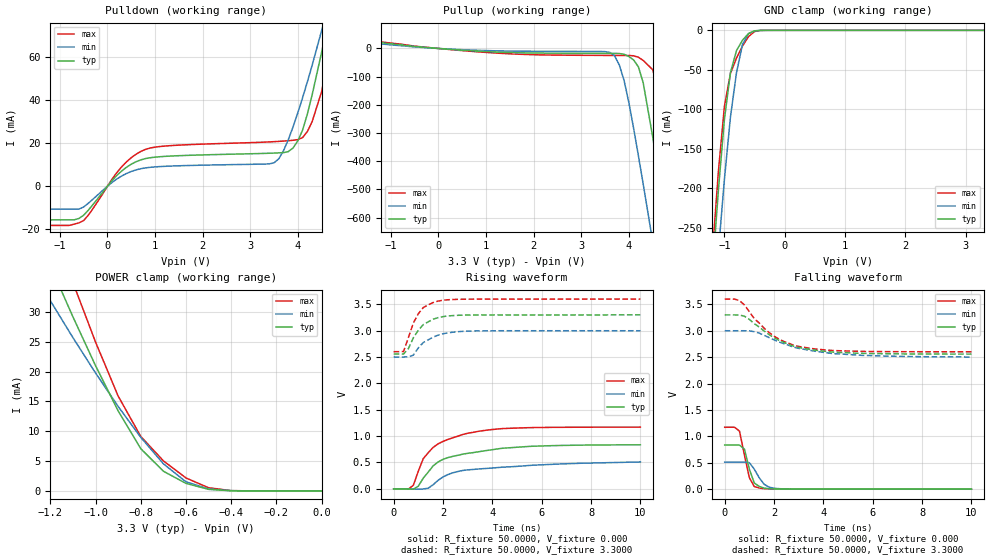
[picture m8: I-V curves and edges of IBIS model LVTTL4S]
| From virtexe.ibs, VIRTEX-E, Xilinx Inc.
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|   Model LVTTL4S
[Model]   LVTTL4S
Model_type   I/O
Polarity   Non-Inverting
Enable   Active-Low
Vinl =   0.800V
Vinh =   2.000V
Vmeas =   1.4000V
Cref =  35.0000pF
Rref =   1.0000M
Vref =  0.000V
C_comp   5.0000pF   4.0000pF   6.0000pF
[Temperature Range]   25.0000   100.0000   0.000
[Voltage Range]   3.3000V   3.0000V   3.6000V
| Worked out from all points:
|   slope of the pulldown table from 0 to 0.495 V, typ, clamps not added: 48.8 ohm
|   slope of the pullup table from 0 to 0.495 V, typ, clamps not added: 80.4 ohm
|   GND clamp passes 1 mA (typ) near -0.51 V on its own axis
|   POWER clamp passes 1 mA (typ) near -0.57 V on its own axis
|   rising waveform, R_fixture 50.0000, V_fixture 0.000: 20-80 % time 1.78ns typ, 2.68ns min, 1.27ns max; typ from 0 V to 0.835 V
|   rising waveform, R_fixture 50.0000, V_fixture 3.3000: 20-80 % time 694ps typ, 820ps min, 587ps max; typ from 2.56 V to 3.3 V
|   falling waveform, R_fixture 50.0000, V_fixture 0.000: 20-80 % time 314ps typ, 436ps min, 320ps max; typ from 0.836 V to 0 V
|   falling waveform, R_fixture 50.0000, V_fixture 3.3000: 20-80 % time 1.65ns typ, 2.15ns min, 1.44ns max; typ from 3.3 V to 2.56 V
[Pulldown]
| voltage   I(typ)   I(min)   I(max)
-3.3V     -15.59mA   -10.6mA    -18.15mA
-700mV    -15.59mA   -10.6mA    -17.58mA
-400mV    -11.06mA   -7.86mA    -13.39mA
300mV     7.091mA    4.771mA    9.036mA
800mV     12.84mA    8.521mA    17.11mA
3.5V      15.39mA    10.89mA    20.68mA
4V        21.07mA    34.12mA    21.62mA
4.2V      33.52mA    48.47mA    25.38mA
4.5V      62.22mA    72.24mA    43.93mA
4.7V      83.65mA    89.14mA    66.44mA
4.9V      106.1mA    106.7mA    91.85mA
6.6V      314.9mA    270.6mA    334.8mA
[Pullup]
| voltage   I(typ)   I(min)   I(max)
-3.3V     66.8mA     64.5mA     64.4mA
-400mV    5.604mA    4.214mA    6.537mA
3.6V      -17.39mA   -14.17mA   -24.69mA
3.8V      -17.91mA   -59.36mA   -24.83mA
3.9V      -20.71mA   -114.4mA   -24.89mA
4.2V      -65.36mA   -380.9mA   -31.21mA
4.3V      -121.5mA   -480.7mA   -42.33mA
4.5V      -313.4mA   -685.2mA   -75.33mA
4.7V      -533.3mA   -893.2mA   -191.1mA
4.9V      -760.6mA   -1.103A    -404.8mA
5.1V      -991.3mA   -1.314A    -635.7mA
6.6V      -2.756A    -2.921A    -2.448A
[GND_clamp]
| voltage   I(typ)   I(min)   I(max)
-3.3V     -2.749A    -2.594A    -2.804A
-1.2V     -306mA     -377.1mA   -282.7mA
-1.1V     -202.5mA   -280mA     -178.8mA
-1V       -112.5mA   -188.5mA   -95.98mA
-900mV    -53.5mA    -109.7mA   -54.53mA
-800mV    -25.67mA   -53.59mA   -35.13mA
-700mV    -12.44mA   -17.88mA   -19.82mA
-600mV    -3.982mA   -4.202mA   -7.865mA
-500mV    -601.5uA   -800.3uA   -1.508mA
-400mV    -51.05uA   -119.3uA   -124.3uA
3.3V      18.74nA    3.634uA    18.92nA
[POWER_clamp]
| voltage   I(typ)   I(min)   I(max)
-3.3V     237mA      175.9mA    284.4mA
-1.3V     46.69mA    38.29mA    56.33mA
-1.2V     37.79mA    31.9mA     45.45mA
-1.1V     29.2mA     25.71mA    34.95mA
-1V       21.01mA    19.78mA    24.97mA
-900mV    13.43mA    14.17mA    15.91mA
-800mV    7.091mA    8.993mA    9.139mA
-700mV    3.305mA    4.554mA    5.052mA
-600mV    1.265mA    1.529mA    2.172mA
-500mV    263.8uA    333.6uA    531.5uA
-400mV    22.63uA    44.12uA    49.77uA
0V        18.8nA     38.3nA     22.53nA
[Ramp]
| variable   typ   min   max
dV/dt_r   0.5010/1.7679n   0.3020/2.5955n   0.7020/1.2208n
dV/dt_f   0.4452/1.6404n   0.2982/2.1491n   0.5988/1.3905n
R_load = 50.0000
[Rising Waveform]
R_fixture = 50.0000
V_fixture = 0.000
| time   V(typ)   V(min)   V(max)
0s        3.793uV    4.235uV    3.708uV
600ps     -4.547mV   -162.8uV   -3.424mV
800ps     -6.325mV   -2.891mV   68.45mV
1ns       50.86mV    -5.707mV   336.6mV
1.2ns     203.2mV    -2.409mV   572.9mV
1.6ns     434.6mV    77.89mV    786.3mV
2.2ns     592.4mV    271mV      937mV
2.8ns     657.6mV    348.3mV    1.031V
4.6ns     776.2mV    415.3mV    1.147V
10ns      835mV      510mV      1.17V
[Rising Waveform]
R_fixture = 50.0000
V_fixture = 3.3000
V_fixture_min = 3.0000
V_fixture_max = 3.6000
| time   V(typ)   V(min)   V(max)
0s        2.557V     2.501V     2.602V
400ps     2.557V     2.501V     2.605V
600ps     2.663V     2.503V     2.872V
800ps     2.866V     2.537V     3.147V
1ns       3.008V     2.673V     3.321V
1.2ns     3.115V     2.775V     3.439V
1.8ns     3.248V     2.916V     3.562V
2.4ns     3.287V     2.971V     3.592V
3.2ns     3.297V     2.994V     3.598V
10ns      3.3V       2.999V     3.6V
[Falling Waveform]
R_fixture = 50.0000
V_fixture = 0.000
| time   V(typ)   V(min)   V(max)
0s        836.4mV    513.6mV    1.172V
400ps     836.4mV    513.6mV    1.173V
600ps     834.6mV    513.6mV    1.099V
800ps     759.3mV    514.1mV    645.6mV
1ns       377.6mV    500.3mV    216.3mV
1.2ns     117.2mV    378.6mV    49.09mV
1.4ns     51.34mV    215mV      22.14mV
1.8ns     8.174mV    37.69mV    5.006mV
2.2ns     2.686mV    9.376mV    2.178mV
10ns      33.84uV    61.14uV    158.6uV
[Falling Waveform]
R_fixture = 50.0000
V_fixture = 3.3000
V_fixture_min = 3.0000
V_fixture_max = 3.6000
| time   V(typ)   V(min)   V(max)
0s        3.3V       3V         3.6V
600ps     3.298V     3V         3.57V
800ps     3.275V     3V         3.49V
1.2ns     3.133V     2.982V     3.229V
1.8ns     2.926V     2.87V      2.965V
2.4ns     2.777V     2.754V     2.797V
3ns       2.683V     2.666V     2.702V
4.4ns     2.595V     2.567V     2.625V
5.6ns     2.571V     2.533V     2.608V
10ns      2.558V     2.503V     2.602V
